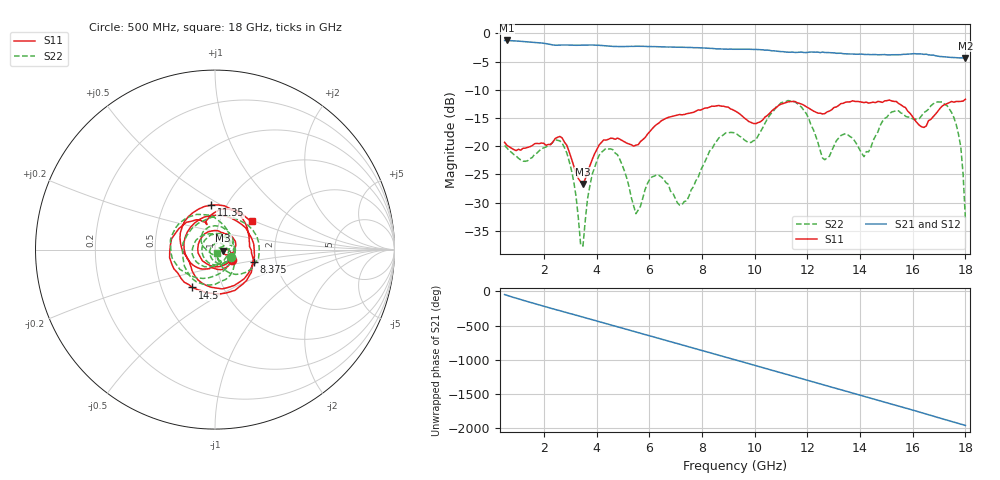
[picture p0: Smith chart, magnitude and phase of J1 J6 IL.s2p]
!Agilent Technologies,N5230A,MY45001360,A.07.50.67
!Agilent N5230A: A.07.50.67
!Date: Tuesday, April 16, 2024 17:41:37
!Correction: S11(Full 2 Port(1,2))
!S21(Full 2 Port(1,2))
!S12(Full 2 Port(1,2))
!S22(Full 2 Port(1,2))
!S2P File: Measurements: S11, S21, S12, S22:
# Hz S  dB  R 50
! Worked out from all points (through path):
!   201 points, 500 MHz to 18 GHz, reference 50 ohm
!   highest |S21| = -1.24 dB at 587.5 MHz (marker M1); lowest = -4.4 dB at 18 GHz (marker M2)
!   group delay of S21, straight-line fit = 302 ps
!   lowest |S11| = -26.7 dB at 3.475 GHz (marker M3), VSWR 1.10, Z = 54.8 - j0.749 ohm
!   |S11| at or under -10 dB: start of sweep to end of sweep
!   |S22| runs from -37.7 to -11.9 dB; largest |S21 - S12| = 0.0081
!   S11 on the Smith chart (normalised r, x): 500 MHz: 1.19, -0.14; 8.375 GHz: 1.53, -0.23; 11.35 GHz: 0.85, +0.45; 14.5 GHz: 0.72, -0.32; 18 GHz: 1.42, +0.49
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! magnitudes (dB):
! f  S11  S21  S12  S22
! 500 MHz  -19.3  -1.2  -1.2  -19.9
! 587.5 MHz  -19.8  -1.2  -1.2  -20.3
! 2.688 GHz  -18.5  -2.0  -2.0  -19.5
! 3.475 GHz  -26.7  -2.1  -2.0  -37.7
! 3.737 GHz  -23.5  -2.0  -2.0  -27.0
! 4.175 GHz  -19.3  -2.1  -2.1  -21.1
! 4.787 GHz  -18.5  -2.3  -2.3  -21.5
! 5.487 GHz  -19.8  -2.3  -2.3  -32.0
! 6.362 GHz  -15.9  -2.4  -2.4  -25.2
! 7.237 GHz  -14.4  -2.4  -2.5  -30.4
! 8.375 GHz  -12.9  -2.6  -2.7  -20.5
! 9.25 GHz  -13.7  -2.8  -2.8  -17.6
! 10.04 GHz  -16.0  -2.8  -2.9  -18.9
! 11.35 GHz  -12.1  -3.3  -3.3  -12.0
! 12.22 GHz  -13.8  -3.3  -3.3  -17.0
! 12.66 GHz  -14.2  -3.4  -3.4  -22.4
! 14.5 GHz  -12.2  -3.7  -3.7  -19.0
! 15.11 GHz  -11.8  -3.8  -3.8  -14.2
! 16.43 GHz  -16.7  -3.7  -3.7  -14.0
! 17.3 GHz  -12.5  -4.2  -4.2  -12.8
! 17.82 GHz  -12.0  -4.3  -4.3  -20.1
! 18 GHz  -11.7  -4.4  -4.4  -32.9
